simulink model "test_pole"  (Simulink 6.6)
settings: Solver=ode45  StartTime=0.0  StopTime=10.0  RelTol=1e-3
libraries: sltpda x3

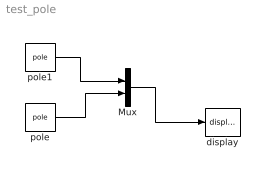
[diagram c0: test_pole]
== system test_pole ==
  Mux : Mux  Inputs=2
  display : sltpda/AO class/display  Tag=display  SystemSampleTime=-1
  pole : sltpda/Modelling/pole  SystemSampleTime=-1  polef=10  poleQ=2
  pole1 : sltpda/Modelling/pole  SystemSampleTime=-1  polef=10
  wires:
  pole/1 -> Mux/2
  pole1/1 -> Mux/1
  Mux/1 -> display/1
